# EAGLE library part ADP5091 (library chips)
Ultralow Power Energy Harvester PMU with MPPT and Charge Management with Backup
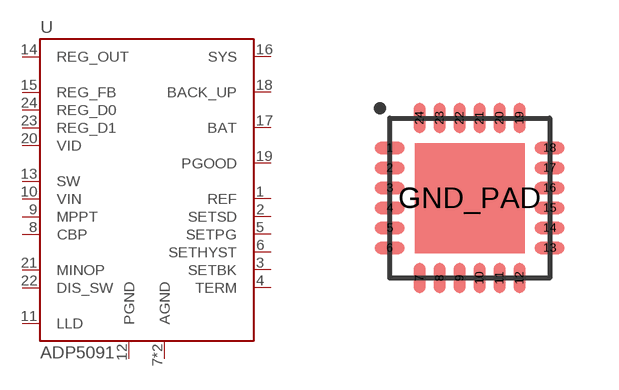
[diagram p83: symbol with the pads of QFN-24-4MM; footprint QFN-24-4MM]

Designator prefix U

## ADP5091 (DIGIKEY: ADP5091ACPZ-1-R7CT-ND; MANUFACTURER: ANALOG DEVICES; MPN: ADP5091ACPZ-1-R7)  [QFN-24-4MM]
1  REF
2  SETSD
3  SETBK
4  TERM
5  SETPG
6  SETHYST
7  AGND
8  CBP
9  MPPT
10  VIN
11  LLD
12  PGND
13  SW
14  REG_OUT
15  REG_FB
16  SYS
17  BAT
18  BACK_UP
19  PGOOD
20  VID
21  MINOP
22  DIS_SW
23  REG_D1
24  REG_D0
GND_PAD  AGND

## Footprint QFN-24-4MM (pad centres in mm)
4mm x 4mm QFN-24
smd 0.75 x 0.3: 1 -2,1.25; 2 -2,0.75; 3 -2,0.25; 4 -2,-0.25; 5 -2,-0.75; 6 -2,-1.25; 13 2,-1.25; 14 2,-0.75; 15 2,-0.25; 16 2,0.25; 17 2,0.75; 18 2,1.25
smd 0.3 x 0.75: 7 -1.25,-2; 8 -0.75,-2; 9 -0.25,-2; 10 0.25,-2; 11 0.75,-2; 12 1.25,-2; 19 1.25,2; 20 0.75,2; 21 0.25,2; 22 -0.25,2; 23 -0.75,2; 24 -1.25,2
smd 2.75 x 2.75: GND_PAD 0,0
